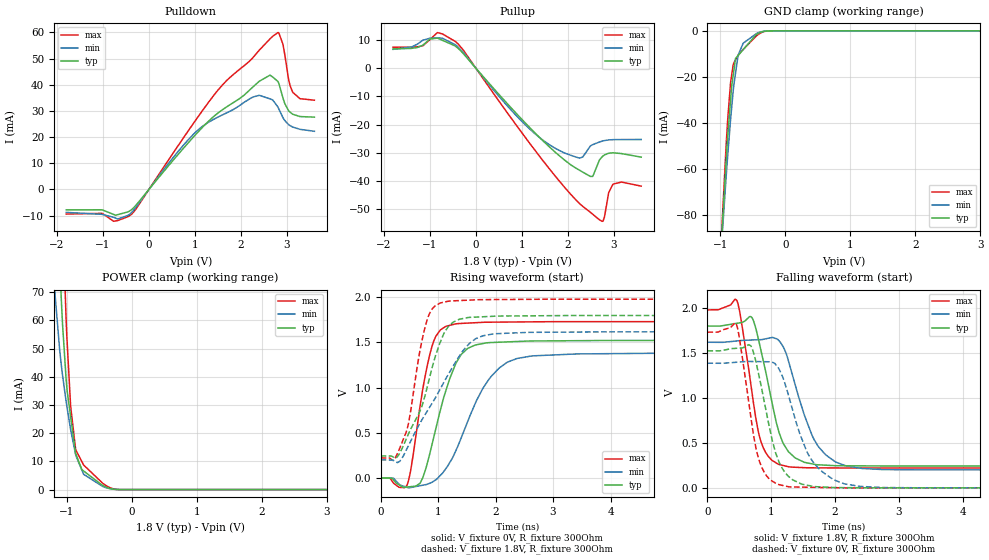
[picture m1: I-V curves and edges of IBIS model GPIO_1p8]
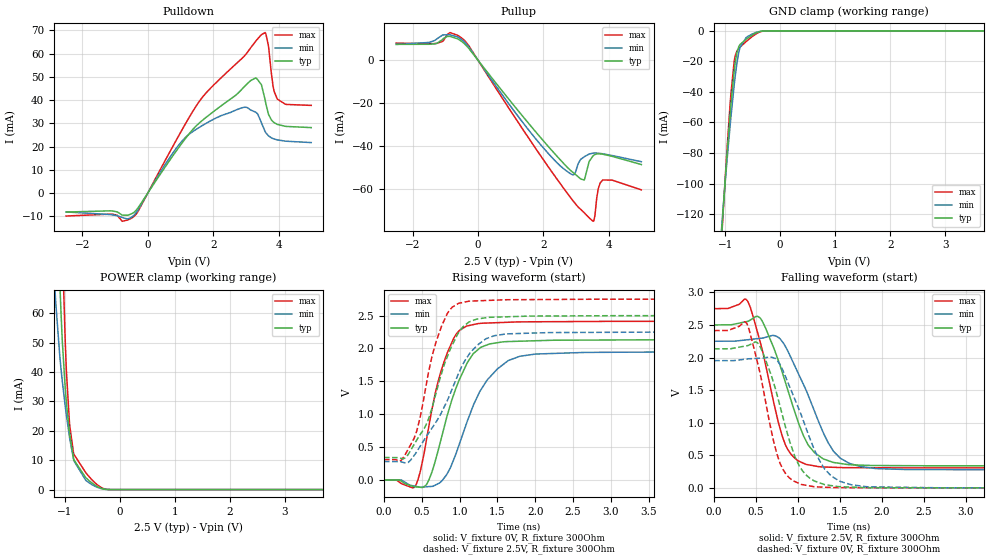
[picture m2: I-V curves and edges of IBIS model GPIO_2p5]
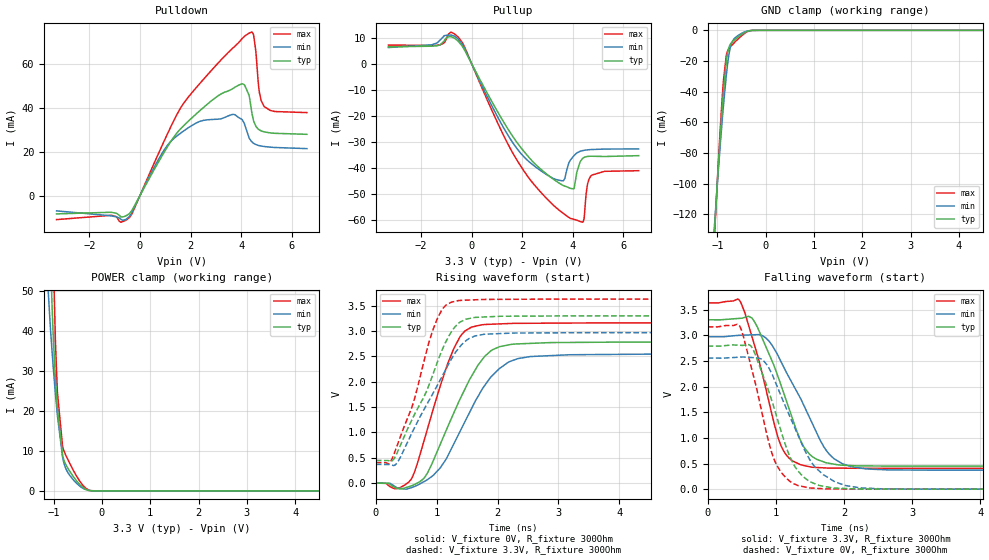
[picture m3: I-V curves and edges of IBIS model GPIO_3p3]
|Texas Instruments Incorporated
| Marketing part#   Digital Voltage Range   Package-type   #pins
|   DP83TC811   1.8V - 3.3V   VQFN   36
[IBIS Ver]   4.1
[File name]   dp83tc811rgm.ibs
[File Rev]   2.0
[Date]   06/21/2019
[Source]
| Texas Instruments Incorporated.
| Analog-eLab Design Center, HPA
| 12500 TI Blvd
| Dallas, TX -75243
[Notes]   Revision History:
| Rev 2.0: 06/21/2019
| - Updated GPIO models and added GPIO1 and GPIO2 models
| Rev 1.0: 08/30/2018
| - Initial version of the model
| - Model generated from simulations in TISPICE
| - C_comp although listed in numerical order of value are
|   obtained from varying PVT conditions. For PVT conditions for
|   each specific value refer the buffer description under
|   respective [Model]. IBIS model user is responsible for using
|   appropriate C_comp to simulate for Signal Integrity.
| - Warnings regarding combined Non-monotonicity of various models have been
|   reviewd and considered minor and can be ignored.
| - Model names with a trailing _1p8 contain the model for 1.8V operation.
|   Model names with a trailing _2p5 contain the model for 2.5V operation.
|   Model names with a trailing _3p3 contain the model for 3.3V operation.
[Disclaimer]
| This model is designed as an aid for customers of Texas Instruments.
| TI and its licensors and suppliers make no warranties, either expressed
| or implied, with respect to this  model, including the warranties of
| merchantability or fitness for a particular purpose. The model is
| provided solely on an "as is" basis. The entire risk as to its quality
| and performance is with the customer.
| This model is subject to change without notice. Texas Instruments
| Incorporated is not responsible for updating this model.
[Copyright]
 (C) Copyright 2019 Texas Instruments Incorporated.All rights reserved.
|   Device
[Component]   DP83TC811
[Manufacturer]   TI
[Package]   |36 VQFN - RND package
|   typ   min   max
R_pkg   0.060   0.048   0.072
L_pkg   0.8nH   0.64nH   0.96nH
C_pkg   0.14pF   0.12pF   0.16pF
[Pin]  signal_name   model_name R_pin  L_pin  C_pin
1   MDC   GPIO   NA   NA   NA
2   INT_N   NC   NA   NA   NA
3   RESET_N   GPIO   NA   NA   NA
4   XO   NC   NA   NA   NA
5   XI   NC   NA   NA   NA
6   LED_1/GPIO_1   GPIO   NA   NA   NA
7   EN   NC   NA   NA   NA
8   WAKE   NC   NA   NA   NA
9   NC   NC   NA   NA   NA
10   INH   NC   NA   NA   NA
11   VDDA   POWER   NA   NA   NA
12   TRD_P   NC   NA   NA   NA
13   TRD_M   NC   NA   NA   NA
14   REX_ER   GPIO   NA   NA   NA
15   RX_DV/CRS_DV/RX_CTRL   GPIO   NA   NA   NA
16   CLKOUT/GPIO_2   GPIO   NA   NA   NA
17   TCK   GPIO   NA   NA   NA
18   TDO   GPIO   NA   NA   NA
19   TMS   GPIO   NA   NA   NA
20   TDI   GPIO   NA   NA   NA
21   NC   NC   NA   NA   NA
22   VDDIO   POWER   NA   NA   NA
23   RX_D3/RX_M   GPIO2   NA   NA   NA
24   RX_D2/RX_P   GPIO2   NA   NA   NA
25   RX_D1/RXCLK_M   GPIO2   NA   NA   NA
26   RX_D0/RXCLK_P   GPIO2   NA   NA   NA
27   RX_CLK   GPIO   NA   NA   NA
28   TX_CLK   GPIO   NA   NA   NA
29   TX_EN/TX_CTRL   GPIO   NA   NA   NA
30   TX_D3   GPIO   NA   NA   NA
31   TX_D2   GPIO   NA   NA   NA
32   TX_D1/TX_P   GPIO1   NA   NA   NA
33   TX_D0/TX_M   GPIO1   NA   NA   NA
34   TX_ER   GPIO   NA   NA   NA
35   LED_0/GPIO_0   GPIO   NA   NA   NA
36   MDIO   GPIO   NA   NA   NA
|   Model Selectors
[Model Selector]  GPIO
GPIO_1p8  GPIO at 1.8V operation
GPIO_2p5  GPIO at 2.5V operation
GPIO_3p3  GPIO at 3.3V operation
[Model Selector]  GPIO1
GPIO1_1p8  GPIO at 1.8V operation
GPIO1_2p5  GPIO at 2.5V operation
GPIO1_3p3  GPIO at 3.3V operation
[Model Selector]  GPIO2
GPIO2_1p8  GPIO at 1.8V operation
GPIO2_2p5  GPIO at 2.5V operation
GPIO2_3p3  GPIO at 3.3V operation
| Models and submodels in the file (9): GPIO_1p8 (I/O), GPIO_2p5 (I/O), GPIO_3p3 (I/O), GPIO1_1p8 (I/O), GPIO1_2p5 (I/O), GPIO1_3p3 (I/O), GPIO2_1p8 (I/O), GPIO2_2p5 (I/O), GPIO2_3p3 (I/O)
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|   GPIO_1p8 Model
[Model]   GPIO_1p8
Model_type   I/O
Polarity   Non-Inverting
Enable   Active-Low
Vinl = 0.63
Vinh = 1.17
Vmeas = 0.9
Vref = 0
Cref = 2pF
Rref = 100000
|   typ   min   max
C_comp   1.4984pF   1.4443pF   1.6131pF
[Model spec]
|subparameter
Vinl   0.63   0.567   0.693
Vinh   1.17   1.053   1.287
| Where Nom  PVT is Nominal Process, 1.8V, 27C
|   Fast PVT is Strong Process,  1.98V, -40C
|   Slow PVT is Weak Process,   1.62V, 125C
[Voltage Range]   1.8   1.62   1.98
|Junction Temperature
[Temperature Range]   27   125   -40
[Pullup Reference]   1.8   1.62   1.98
[Pulldown Reference]   0   0   0
[Power Clamp Reference]   1.8   1.62   1.98
[GND Clamp Reference]   0   0   0
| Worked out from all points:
|   slope of the pulldown table from 0 to 0.27 V, typ, clamps not added: 46.9 ohm
|   slope of the pullup table from 0 to 0.27 V, typ, clamps not added: 53.6 ohm
|   GND clamp passes 1 mA (typ) near -0.41 V on its own axis
|   POWER clamp passes 1 mA (typ) near -0.41 V on its own axis
|   falling waveform, V_fixture 1.8V, R_fixture 300Ohm: 20-80 % time 303ps typ, 416ps min, 235ps max; typ from 1.8 V to 0.243 V
|   rising waveform, V_fixture 0V, R_fixture 300Ohm: 20-80 % time 409ps typ, 614ps min, 277ps max; typ from 0 V to 1.52 V
|   rising waveform, V_fixture 1.8V, R_fixture 300Ohm: 20-80 % time 493ps typ, 773ps min, 284ps max; typ from 0.243 V to 1.8 V
|   falling waveform, V_fixture 0V, R_fixture 300Ohm: 20-80 % time 297ps typ, 430ps min, 233ps max; typ from 1.52 V to 0 V
[Pulldown]
|   Voltage   I(typ)   I(min)   I(max)
-1.8V     -7.815mA   -8.783mA   -9.427mA
-1.012V   -7.855mA   -9.578mA   -9.226mA
-768.6mV  -9.565mA   -10.68mA   -12.2mA
-390.6mV  -7.919mA   -9.076mA   -9.66mA
1.165V    23.73mA    24.11mA    30.11mA
2.401V    41.32mA    35.95mA    53.21mA
2.633V    43.65mA    34.6mA     57.5mA
2.806V    41.24mA    31.48mA    59.92mA
2.914V    35.03mA    27.45mA    55.52mA
3.038V    30.09mA    24.77mA    42.01mA
3.125V    28.76mA    23.85mA    37.24mA
3.6V      27.61mA    22.2mA     34.08mA
[GND Clamp]
|   Voltage   I(typ)   I(min)   I(max)
-1.8V     -586.6mA   -535.7mA   -625.9mA
-1.001V   -99.27mA   -100.5mA   -98.41mA
-914.4mV  -57.62mA   -64.38mA   -50.86mA
-887.4mV  -45.87mA   -54.01mA   -38.3mA
-844.2mV  -30.18mA   -38.65mA   -22.58mA
-806.4mV  -19.85mA   -26.91mA   -15.17mA
-768.6mV  -12.06mA   -18.59mA   -12.69mA
-725.4mV  -10.65mA   -10.42mA   -10.58mA
-649.8mV  -8.179mA   -5.383mA   -8.069mA
-444.6mV  -1.565mA   -1.167mA   -2.19mA
-212.4mV  -18.11uA   -20.42uA   -20.45uA
3.6V      0A         0A         0A
[Pullup]
|   Voltage   I(typ)   I(min)   I(max)
-1.8V     6.759mA    6.611mA    7.381mA
-1.152V   8.09mA     9.847mA    7.887mA
-833.4mV  10.6mA     10.7mA     12.56mA
-444.6mV  7.764mA    8.247mA    9.418mA
856.8mV   -15.62mA   -16.4mA    -19.66mA
1.618V    -28.14mA   -27.29mA   -36mA
2.266V    -36.24mA   -31.86mA   -48.1mA
2.493V    -38.34mA   -27.58mA   -51.03mA
2.747V    -31.46mA   -25.88mA   -54.24mA
2.893V    -30.13mA   -25.44mA   -44.04mA
2.984V    -29.99mA   -25.34mA   -41.14mA
3.6V      -31.53mA   -25.29mA   -41.79mA
[POWER Clamp]
|   Voltage   I(typ)   I(min)   I(max)
-1.8V     670.8mA    497.2mA    807.9mA
-1.184V   129.3mA    70.13mA    198.4mA
-1.087V   68.67mA    44.65mA    114.6mA
-1.066V   58.56mA    40.52mA    97.74mA
-1.012V   39.41mA    31.41mA    60.89mA
-995.4mV  35.1mA     28.97mA    52.43mA
-941.4mV  25.86mA    21.28mA    29.56mA
-860.4mV  12.59mA    12.01mA    13.99mA
-741.6mV  6.6mA      5.425mA    8.724mA
-444.6mV  1.42mA     1.065mA    2.177mA
-180mV    12.05uA    16.39uA    15.62uA
3.6V      0A         0A         0A
[Ramp]
R_load = 300
|   typ   min   max
dV/dt_r   0.914841/4.05292e-10   0.832077/6.12912e-10   1.03915/2.7572e-10
dV/dt_f   0.934002/3.00042e-10   0.852202/4.14261e-10   1.05541/2.34847e-10
[Falling Waveform]
V_fixture = 1.8V
V_fixture_min = 1.62V
V_fixture_max = 1.98V
R_fixture = 300Ohm
C_fixture = 0F
|   Time   V(typ)   V(min)   V(max)
0s        1.8V       1.62V      1.98V
457.5ps   1.83V      1.634V     2.088V
701.9ps   1.889V     1.645V     1.041V
798.6ps   1.655V     1.648V     621.9mV
909ps     1.305V     1.657V     397.4mV
1.123ns   613mV      1.635V     260.2mV
1.27ns    401.4mV    1.41V      234.9mV
1.734ns   256.7mV    464mV      222.6mV
2.427ns   244.7mV    215.5mV    221.1mV
20ns      243.3mV    199.6mV    220.9mV
[Rising Waveform]
V_fixture = 0V
V_fixture_min = 0V
V_fixture_max = 0V
R_fixture = 300Ohm
C_fixture = 0F
|   Time   V(typ)   V(min)   V(max)
0s        27.87uV    64.48uV    36.63uV
457.5ps   -100.9mV   -104.9mV   -82.66mV
525.4ps   -96.57mV   -106.3mV   93.37mV
688.3ps   -55.99mV   -86.35mV   802.6mV
927.8ps   459.2mV    -34.36mV   1.521V
1.296ns   1.248V     283.3mV    1.705V
1.519ns   1.436V     630.8mV    1.715V
1.906ns   1.499V     1.11V      1.725V
2.66ns    1.517V     1.352V     1.729V
20ns      1.525V     1.387V     1.732V
[Rising Waveform]
V_fixture = 1.8V
V_fixture_min = 1.62V
V_fixture_max = 1.98V
R_fixture = 300Ohm
C_fixture = 0F
|   Time   V(typ)   V(min)   V(max)
0s        243.3mV    199.6mV    220.9mV
302.6ps   245.8mV    172.4mV    281.8mV
481.2ps   482.8mV    353mV      594.1mV
675.8ps   727.9mV    595.3mV    1.38V
813ps     1.012V     741.5mV    1.759V
1.026ns   1.487V     972.7mV    1.933V
1.175ns   1.674V     1.143V     1.957V
1.656ns   1.781V     1.542V     1.972V
2.569ns   1.795V     1.612V     1.978V
20ns      1.8V       1.62V      1.98V
[Falling Waveform]
|Gnd
V_fixture = 0V
V_fixture_min = 0V
V_fixture_max = 0V
R_fixture = 300Ohm
C_fixture = 0F
|   Time   V(typ)   V(min)   V(max)
0s        1.525V     1.387V     1.732V
450.8ps   1.552V     1.397V     1.825V
682.1ps   1.577V     1.406V     776.5mV
764.7ps   1.387V     1.405V     426.4mV
887.7ps   968.4mV    1.404V     176.1mV
1.067ns   391.6mV    1.374V     52.85mV
1.27ns    127.5mV    1.029V     12.46mV
1.661ns   15.96mV    282.1mV    6.055mV
2.398ns   1.206mV    16.02mV    167.4uV
20ns      27.35uV    63.74uV    36.67uV
|   GPIO_2p5 Model
[Model]   GPIO_2p5
Model_type   I/O
Polarity   Non-Inverting
Enable   Active-Low
Vinl = 0.7
Vinh = 1.7
Vmeas = 1.25
Vref = 0
Cref = 2pF
Rref = 100000
|   typ   min   max
C_comp   1.4643pF   1.3920pF   1.5691pF
| Where Nom  PVT is Nominal Process, 2.5V, 27C
|   Fast PVT is Strong Process,  2.75V, -40C
|   Slow PVT is Weak Process,   2.25V, 125C
[Voltage Range]   2.5   2.25   2.75
|Junction Temperature
[Temperature Range]   27   125   -40
[Pullup Reference]   2.5   2.25   2.75
[Pulldown Reference]   0   -0   0
[Power Clamp Reference]   2.5   2.25   2.75
[GND Clamp Reference]   0   0   0
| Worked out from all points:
|   slope of the pulldown table from 0 to 0.375 V, typ, clamps not added: 47.1 ohm
|   slope of the pullup table from 0 to 0.375 V, typ, clamps not added: 51.4 ohm
|   GND clamp passes 1 mA (typ) near -0.41 V on its own axis
|   POWER clamp passes 1 mA (typ) near -0.41 V on its own axis
|   falling waveform, V_fixture 2.5V, R_fixture 300Ohm: 20-80 % time 343ps typ, 402ps min, 268ps max; typ from 2.5 V to 0.339 V
|   rising waveform, V_fixture 0V, R_fixture 300Ohm: 20-80 % time 359ps typ, 449ps min, 294ps max; typ from 0 V to 2.13 V
|   rising waveform, V_fixture 2.5V, R_fixture 300Ohm: 20-80 % time 384ps typ, 526ps min, 293ps max; typ from 0.339 V to 2.5 V
|   falling waveform, V_fixture 0V, R_fixture 300Ohm: 20-80 % time 296ps typ, 373ps min, 243ps max; typ from 2.13 V to 0 V
[Pulldown]
|   Voltage   I(typ)   I(min)   I(max)
-2.5V     -8.189mA   -8.135mA   -9.9mA
-407.5mV  -8.128mA   -9.347mA   -9.894mA
852.5mV   17.75mA    18.92mA    22.3mA
1.482V    28.92mA    27.44mA    37.52mA
2.848V    44.21mA    36.54mA    57.52mA
3.305V    49.58mA    34.76mA    65.42mA
3.478V    46.54mA    30.19mA    68.2mA
3.59V     40.06mA    26.43mA    69.07mA
3.695V    33.83mA    24.6mA     62.93mA
3.83V     30.71mA    23.45mA    46.18mA
3.958V    29.58mA    22.89mA    40.56mA
5V        28.16mA    21.72mA    37.72mA
[GND Clamp]
|   Voltage   I(typ)   I(min)   I(max)
-2.5V     -1.034A    -947.3mA   -1.104A
-1.113V   -161.2mA   -152.9mA   -167.3mA
-1.038V   -118.9mA   -117mA     -120.5mA
-962.5mV  -79.76mA   -83.97mA   -76.34mA
-910mV    -55.2mA    -62.66mA   -48.71mA
-827.5mV  -24.15mA   -33.23mA   -18.53mA
-782.5mV  -13.95mA   -20.65mA   -13.08mA
-730mV    -9.039mA   -10.98mA   -10.75mA
-617.5mV  -5.455mA   -4.423mA   -7.047mA
-497.5mV  -2.593mA   -1.97mA    -3.519mA
-197.5mV  -12.52uA   -15.34uA   -17.8uA
5V        0A         0A         0A
[Pullup]
|   Voltage   I(typ)   I(min)   I(max)
-2.5V     7.343mA    7.313mA    7.913mA
-1.255V   7.831mA    9.881mA    7.795mA
-857.5mV  11.08mA    11.79mA    12.83mA
-452.5mV  8.165mA    8.997mA    9.734mA
2.533V    -46.63mA   -49.43mA   -57.79mA
2.93V     -52.54mA   -53.41mA   -65.88mA
3.252V    -55.8mA    -44.99mA   -71.05mA
3.522V    -44.55mA   -43.3mA    -75.04mA
3.575V    -44.01mA   -43.27mA   -72.81mA
3.68V     -43.64mA   -43.34mA   -59.91mA
3.815V    -43.79mA   -43.6mA    -55.87mA
5V        -48.62mA   -47.3mA    -60.4mA
[POWER Clamp]
|   Voltage   I(typ)   I(min)   I(max)
-2.5V     1.336A     1.089A     1.531A
-1.173V   120.8mA    65.99mA    187.7mA
-1.083V   66.33mA    43.57mA    110.8mA
-1.045V   50.26mA    36.74mA    82.68mA
-992.5mV  34.39mA    28.38mA    50.31mA
-970mV    29.3mA     25.1mA     39.83mA
-917.5mV  19.8mA     18.15mA    23.26mA
-842.5mV  10.72mA    10.39mA    12.48mA
-617.5mV  4.019mA    3.114mA    5.71mA
-445mV    1.425mA    1.073mA    2.195mA
-145mV    6.667uA    8.378uA    11.54uA
5V        0A         0A         0A
[Ramp]
R_load = 300
|   typ   min   max
dV/dt_r   1.28023/3.56144e-10   1.17216/4.45927e-10   1.44785/2.93944e-10
dV/dt_f   1.29669/3.40592e-10   1.18281/4.01879e-10   1.46551/2.67366e-10
[Falling Waveform]
V_fixture = 2.5V
V_fixture_min = 2.25V
V_fixture_max = 2.75V
R_fixture = 300Ohm
C_fixture = 0F
|   Time   V(typ)   V(min)   V(max)
0s        2.5V       2.25V      2.75V
379.6ps   2.549V     2.27V      2.893V
554ps     2.599V     2.295V     2.219V
735.5ps   2.065V     2.332V     1.177V
857.9ps   1.591V     2.152V     641.1mV
1.066ns   800.5mV    1.586V     378.2mV
1.246ns   496.2mV    1.021V     325.9mV
1.506ns   374.6mV    455.1mV    312mV
1.961ns   342.6mV    294mV      308.2mV
20ns      338.8mV    278.6mV    307.4mV
[Rising Waveform]
V_fixture = 0V
V_fixture_min = 0V
V_fixture_max = 0V
R_fixture = 300Ohm
C_fixture = 0F
|   Time   V(typ)   V(min)   V(max)
0s        59.48uV    69.67uV    139.9uV
395.8ps   -104.8mV   -93.55mV   -118.6mV
473.9ps   -113.2mV   -111.4mV   99.06mV
563.1ps   -69.76mV   -105.9mV   615.7mV
717.7ps   451.4mV    -57.88mV   1.504V
922.6ps   1.298V     310.2mV    2.155V
1.246ns   1.984V     1.292V     2.378V
1.645ns   2.104V     1.816V     2.398V
2.655ns   2.126V     1.939V     2.409V
20ns      2.134V     1.954V     2.413V
[Rising Waveform]
V_fixture = 2.5V
V_fixture_min = 2.25V
V_fixture_max = 2.75V
R_fixture = 300Ohm
C_fixture = 0F
|   Time   V(typ)   V(min)   V(max)
0s        338.8mV    278.6mV    307.4mV
321ps     386.1mV    265.8mV    467.4mV
433.9ps   606.3mV    429.2mV    744.3mV
571.7ps   874.9mV    679.9mV    1.528V
766.7ps   1.639V     1.039V     2.352V
902.8ps   2.05V      1.386V     2.627V
1.118ns   2.397V     1.898V     2.718V
1.459ns   2.475V     2.193V     2.734V
2.185ns   2.493V     2.241V     2.744V
20ns      2.5V       2.25V      2.75V
[Falling Waveform]
|Gnd
V_fixture = 0V
V_fixture_min = 0V
V_fixture_max = 0V
R_fixture = 300Ohm
C_fixture = 0F
|   Time   V(typ)   V(min)   V(max)
0s        2.133V     1.952V     2.413V
375.3ps   2.177V     1.974V     2.545V
527.1ps   2.212V     1.988V     1.876V
700.6ps   1.651V     1.998V     766.9mV
789.2ps   1.242V     1.885V     370.7mV
964.3ps   479.6mV    1.356V     96.73mV
1.188ns   110.7mV    611.8mV    18.73mV
1.403ns   34.14mV    176mV      5.38mV
1.84ns    3.507mV    15.95mV    1.39mV
20ns      58.22uV    68.87uV    135.8uV
|   GPIO_3p3 Model
[Model]   GPIO_3p3
Model_type   I/O
Polarity   Non-Inverting
Enable   Active-Low
Vinl = 0.8
Vinh = 2
Vmeas = 1.65
Vref = 0
Cref = 2pF
Rref = 100000
|   typ   min   max
C_comp   1.3729pF   1.3355pF   1.4443pF
| Where Nom  PVT is Nominal Process, 3.3V, 27C
|   Fast PVT is Strong Process,  3.63V, -40C
|   Slow PVT is Weak Process,   2.97V, 125C
[Voltage Range]   3.3   2.97   3.63
|Junction Temperature
[Temperature Range]   27   125   -40
[Pullup Reference]   3.3   2.97   3.63
[Pulldown Reference]   0   0   -0
[Power Clamp Reference]   3.3   2.97   3.63
[GND Clamp Reference]   0   0   0
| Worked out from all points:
|   slope of the pulldown table from 0 to 0.495 V, typ, clamps not added: 47.3 ohm
|   slope of the pullup table from 0 to 0.495 V, typ, clamps not added: 54.4 ohm
|   GND clamp passes 1 mA (typ) near -0.41 V on its own axis
|   POWER clamp passes 1 mA (typ) near -0.41 V on its own axis
|   falling waveform, V_fixture 3.3V, R_fixture 300Ohm: 20-80 % time 472ps typ, 588ps min, 376ps max; typ from 3.3 V to 0.449 V
|   rising waveform, V_fixture 0V, R_fixture 300Ohm: 20-80 % time 648ps typ, 689ps min, 497ps max; typ from 0 V to 2.79 V
|   rising waveform, V_fixture 3.3V, R_fixture 300Ohm: 20-80 % time 624ps typ, 689ps min, 483ps max; typ from 0.449 V to 3.3 V
|   falling waveform, V_fixture 0V, R_fixture 300Ohm: 20-80 % time 427ps typ, 524ps min, 352ps max; typ from 2.79 V to 0 V
[Pulldown]
|   Voltage   I(typ)   I(min)   I(max)
-3.3V     -8.393mA   -7.01mA    -10.99mA
-429mV    -8.362mA   -9.656mA   -10.16mA
986.7mV   20.38mA    21.38mA    25.7mA
1.957V    34.48mA    31.35mA    45.66mA
3.759V    49.57mA    37mA       68.34mA
4.125V    50.73mA    33.04mA    72.75mA
4.343V    44.18mA    25.81mA    74.44mA
4.501V    33.93mA    23.85mA    72.94mA
4.58V     31.77mA    23.36mA    66.24mA
4.719V    30.06mA    22.84mA    47.64mA
4.907V    29.14mA    22.44mA    40.78mA
6.6V      28.01mA    21.47mA    37.94mA
[GND Clamp]
|   Voltage   I(typ)   I(min)   I(max)
-3.3V     -1.55A     -1.423A    -1.652A
-1.063V   -132.8mA   -128.7mA   -135.9mA
-1.003V   -100.5mA   -101.5mA   -99.83mA
-943.8mV  -70.69mA   -76.2mA    -66.07mA
-894.3mV  -48.46mA   -56.62mA   -41.35mA
-874.5mV  -40.43mA   -49.25mA   -32.94mA
-815.1mV  -20.72mA   -29.44mA   -16.34mA
-765.6mV  -11.73mA   -16.89mA   -12.16mA
-706.2mV  -8.023mA   -8.475mA   -9.925mA
-636.9mV  -5.964mA   -4.966mA   -7.658mA
-419.1mV  -1.13mA    -855.6uA   -1.634mA
6.6V      0A         0A         0A
[Pullup]
|   Voltage   I(typ)   I(min)   I(max)
-3.3V     6.638mA    6.338mA    7.299mA
-1.251V   7.371mA    9.234mA    7.347mA
-587.4mV  9.173mA    9.996mA    10.78mA
2.026V    -33.08mA   -35.23mA   -40.5mA
3.6V      -46.52mA   -44.81mA   -57.17mA
3.897V    -47.69mA   -36.86mA   -59.18mA
4.046V    -47.73mA   -35.1mA    -59.58mA
4.155V    -41.43mA   -34.12mA   -59.91mA
4.412V    -35.98mA   -33.14mA   -60.41mA
4.571V    -35.45mA   -32.92mA   -46.39mA
4.749V    -35.36mA   -32.78mA   -42.59mA
6.6V      -35.14mA   -32.55mA   -40.92mA
[POWER Clamp]
|   Voltage   I(typ)   I(min)   I(max)
-3.3V     2.109A     1.785A     2.366A
-1.112V   82.02mA    49.75mA    135mA
-1.063V   57.26mA    39.83mA    95.49mA
-1.033V   45.98mA    34.71mA    74.36mA
-1.003V   37.11mA    29.99mA    56.06mA
-963.6mV  27.98mA    24.2mA     37.24mA
-924mV    20.83mA    18.95mA    24.8mA
-815.1mV  8.873mA    8.438mA    10.98mA
-755.7mV  6.746mA    5.802mA    9.104mA
-676.5mV  5.088mA    4.045mA    7.098mA
-339.9mV  432.6uA    346.4uA    736.9uA
6.6V      0A         0A         0A
[Ramp]
R_load = 300
|   typ   min   max
dV/dt_r   1.67353/6.43576e-10   1.53376/6.86094e-10   1.89789/4.93352e-10
dV/dt_f   1.71076/4.71962e-10   1.55992/5.88452e-10   1.93409/3.76098e-10
[Falling Waveform]
V_fixture = 3.3V
V_fixture_min = 2.97V
V_fixture_max = 3.63V
R_fixture = 300Ohm
C_fixture = 0F
|   Time   V(typ)   V(min)   V(max)
0s        3.3V       2.97V      3.63V
457.8ps   3.327V     2.997V     3.693V
662.9ps   3.31V      3.007V     2.913V
871.5ps   2.722V     2.925V     1.857V
1.076ns   2.028V     2.485V     845.4mV
1.358ns   965.3mV    1.782V     479.1mV
1.522ns   650.3mV    1.319V     429.2mV
1.857ns   486.8mV    591.3mV    410.1mV
2.649ns   450mV      375.5mV    406.5mV
20ns      448.6mV    370mV      406.3mV
[Rising Waveform]
V_fixture = 0V
V_fixture_min = 0V
V_fixture_max = 0V
R_fixture = 300Ohm
C_fixture = 0F
|   Time   V(typ)   V(min)   V(max)
0s        25.31uV    64.17uV    17.36uV
540.7ps   -69.46mV   -104.6mV   20.93mV
784.7ps   89.34mV    25.94mV    808.3mV
1.056ns   759.7mV    298mV      1.907V
1.285ns   1.396V     785.5mV    2.665V
1.465ns   1.86V      1.216V     3.002V
1.733ns   2.411V     1.822V     3.12V
2.193ns   2.729V     2.394V     3.147V
3.184ns   2.774V     2.532V     3.157V
20ns      2.789V     2.556V     3.163V
[Rising Waveform]
V_fixture = 3.3V
V_fixture_min = 2.97V
V_fixture_max = 3.63V
R_fixture = 300Ohm
C_fixture = 0F
|   Time   V(typ)   V(min)   V(max)
0s        448.6mV    370mV      406.3mV
208.5ps   443.6mV    368mV      381.6mV
306ps     494.2mV    352.2mV    598.6mV
613.2ps   1.302V     1.042V     1.576V
995ps     2.335V     1.895V     3.2V
1.143ns   2.771V     2.23V      3.5V
1.354ns   3.145V     2.649V     3.599V
1.63ns    3.268V     2.902V     3.615V
2.262ns   3.292V     2.96V      3.625V
20ns      3.3V       2.97V      3.63V
[Falling Waveform]
|Gnd
V_fixture = 0V
V_fixture_min = 0V
V_fixture_max = 0V
R_fixture = 300Ohm
C_fixture = 0F
|   Time   V(typ)   V(min)   V(max)
0s        2.789V     2.554V     3.163V
450.2ps   2.805V     2.571V     3.206V
638ps     2.783V     2.565V     2.384V
820ps     2.185V     2.502V     1.349V
995ps     1.492V     2.082V     519.3mV
1.259ns   487.6mV    1.255V     108.7mV
1.489ns   156.4mV    595.4mV    24.42mV
1.873ns   21.1mV     141.7mV    3.957mV
2.568ns   1.916mV    5.909mV    300.7uV
20ns      25.01uV    64.25uV    17.87uV
